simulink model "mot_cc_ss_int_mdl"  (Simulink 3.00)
settings: Solver=ode45  StartTime=0.0  StopTime=10.0  RelTol=1e-6  AbsTol=1e-6
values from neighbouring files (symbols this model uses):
  b = Ic0*Ke/Wmax    (= 8.2054202412e-06)    [mot_cc_ss_int.m]    (also in mot_cc_ss_k.m; Regolatore_Rs_discreto.m = -h*alpha; mot_cc_ss.m)
  C0 = 0*N*m    (= 0)    [mot_cc_ss_int.m]    (also in mot_cc_ss_k.m; mot_cc_ss.m)
  Ia0 = 0    [mot_cc_ss_int.m]    (also in mot_cc_ss_k.m; mot_cc_ss.m)
  Ia_max = Imax    (= 93.6)    [mot_cc_ss_int.m]    (also in mot_cc_ss_k.m)
  J = 9.2775e-006    (= 9.2775e-06)    [mot_cc_ss_int.m]    (also in mot_cc_ss_k.m; mot_cc_ss.m)
  K = (1-perc)/(perc*evalfr(G1s,0))    [mot_cc_ss_int.m]    (also in mot_cc_ss_k.m = K_sigma)
  Ke = Cmax/Imax    (= 0.00651965811966)    [mot_cc_ss_int.m]    (also in mot_cc_ss_k.m; mot_cc_ss.m)
  L = 60*10^-6    (= 6e-05)    [mot_cc_ss_int.m]    (also in mot_cc_ss_k.m; mot_cc_ss.m)
  R = Vn/Imax    (= 0.128205128205)    [mot_cc_ss_int.m]    (also in mot_cc_ss_k.m; mot_cc_ss.m)
  tau1 = (M-cos(phi))/(wa*sin(phi))    [mot_cc_ss_int.m]    (also in Regolatore_Rs_discreto.m = 0.806)
  tau2 = (cos(phi)-1/M)/(wa*sin(phi))    [mot_cc_ss_int.m]    (also in Regolatore_Rs_discreto.m = 0.117)
  Tcsim = T_sim/1000    (= 8.42051458616e-06)    [mot_cc_ss_int.m]    (also in mot_cc_ss_k.m = 0.0001; mot_cc_ss.m = 0.001)
  Th0 = 0    [mot_cc_ss_int.m]    (also in mot_cc_ss_k.m; mot_cc_ss.m)
  Vi_max = Vn    (= 12)    [mot_cc_ss_int.m]    (also in mot_cc_ss_k.m)
  W_ref = R0    (= 100)    [mot_cc_ss_int.m]    (also in mot_cc_ss_k.m = 1047.1975512)
  Wm0 = 0    [mot_cc_ss_int.m]    (also in mot_cc_ss_k.m; mot_cc_ss.m)

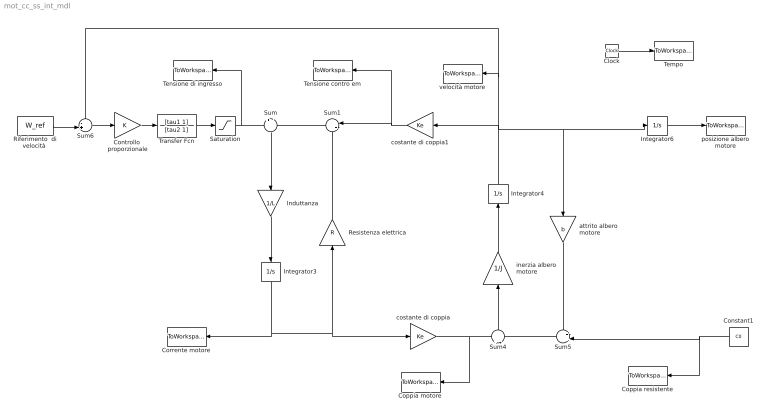
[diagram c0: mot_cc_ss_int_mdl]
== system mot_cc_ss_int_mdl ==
  Clock : Clock
  Constant1 : Constant  Orientation=left  Value=C0
  Controllo  proporzionale : Gain  Gain=K  SaturateOnIntegerOverflow=on
  Coppia motore : ToWorkspace  VariableName=Cm  SampleTime=Tcsim  SaveFormat=Matrix
  Coppia resistente : ToWorkspace  VariableName=Cr  SampleTime=Tcsim  SaveFormat=Matrix
  Corrente motore : ToWorkspace  VariableName=Ia  SampleTime=Tcsim  SaveFormat=Matrix
  Induttanza : Gain  Orientation=down  Gain=1/L  SaturateOnIntegerOverflow=on
  Integrator3 : Integrator  Orientation=down  ExternalReset=none  InitialConditionSource=internal  InitialCondition=Ia0  LimitOutput=on  UpperSaturationLimit=Ia_max  LowerSaturationLimit=-Ia_max  ShowSaturationPort=off  ShowStatePort=off  AbsoluteTolerance=auto
  Integrator4 : Integrator  Orientation=up  ExternalReset=none  InitialConditionSource=internal  InitialCondition=Wm0  LimitOutput=off  UpperSaturationLimit=inf  LowerSaturationLimit=-inf  ShowSaturationPort=off  ShowStatePort=off  AbsoluteTolerance=auto
  Integrator6 : Integrator  ExternalReset=none  InitialConditionSource=internal  InitialCondition=Th0  LimitOutput=off  UpperSaturationLimit=inf  LowerSaturationLimit=-inf  ShowSaturationPort=off  ShowStatePort=off  AbsoluteTolerance=auto
  Resistenza elettrica : Gain  Orientation=up  Gain=R  SaturateOnIntegerOverflow=on
  "Riferimento  di velocità " : Constant  Value=W_ref
  Saturation : Saturate  UpperLimit=Vi_max  LowerLimit=-Vi_max
  Sum : Sum  Orientation=down  Inputs=+|-  SaturateOnIntegerOverflow=on
  Sum1 : Sum  Orientation=left  Inputs=|++  SaturateOnIntegerOverflow=on
  Sum4 : Sum  Orientation=up  Inputs=+|-  SaturateOnIntegerOverflow=on
  Sum5 : Sum  Orientation=left  Inputs=++|  SaturateOnIntegerOverflow=on
  Sum6 : Sum  Inputs=-+|  SaturateOnIntegerOverflow=on
  Tempo : ToWorkspace  VariableName=t  SampleTime=Tcsim  SaveFormat=Matrix
  Tensione contro em : ToWorkspace  VariableName=E  SampleTime=Tcsim  SaveFormat=Matrix
  Tensione di ingresso : ToWorkspace  VariableName=Vi  SampleTime=Tcsim  SaveFormat=Matrix
  Transfer Fcn : TransferFcn  Numerator=[tau1 1]  Denominator=[tau2 1]
  attrito albero motore : Gain  Orientation=down  Gain=b  SaturateOnIntegerOverflow=on
  costante di coppia : Gain  Gain=Ke  SaturateOnIntegerOverflow=on
  costante di coppia1 : Gain  Orientation=left  Gain=Ke  SaturateOnIntegerOverflow=on
  inerzia albero motore : Gain  Orientation=up  Gain=1/J  SaturateOnIntegerOverflow=on
  posizione albero motore : ToWorkspace  VariableName=Th  SampleTime=Tcsim  SaveFormat=Matrix
  velocità motore : ToWorkspace  VariableName=Wm  SampleTime=Tcsim  SaveFormat=Matrix
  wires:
  Sum/1 -> Induttanza/1
  Induttanza/1 -> Integrator3/1
  Sum1/1 -> Sum/2
  Integrator3/1 -> Corrente motore/1, costante di coppia/1, Resistenza elettrica/1
  Resistenza elettrica/1 -> Sum1/2
  Sum4/1 -> inerzia albero motore/1
  inerzia albero motore/1 -> Integrator4/1
  Sum5/1 -> Sum4/2
  attrito albero motore/1 -> Sum5/1
  Constant1/1 -> Coppia resistente/1, Sum5/2
  Integrator4/1 -> costante di coppia1/1, attrito albero motore/1, Integrator6/1, velocità motore/1, Sum6/1
  Integrator6/1 -> posizione albero motore/1
  costante di coppia/1 -> Sum4/1, Coppia motore/1
  costante di coppia1/1 -> Sum1/1, Tensione contro em/1
  Clock/1 -> Tempo/1
  Sum6/1 -> Controllo  proporzionale/1
  Saturation/1 -> Sum/1, Tensione di ingresso/1
  "Riferimento  di velocità "/1 -> Sum6/2
  Controllo  proporzionale/1 -> Transfer Fcn/1
  Transfer Fcn/1 -> Saturation/1
